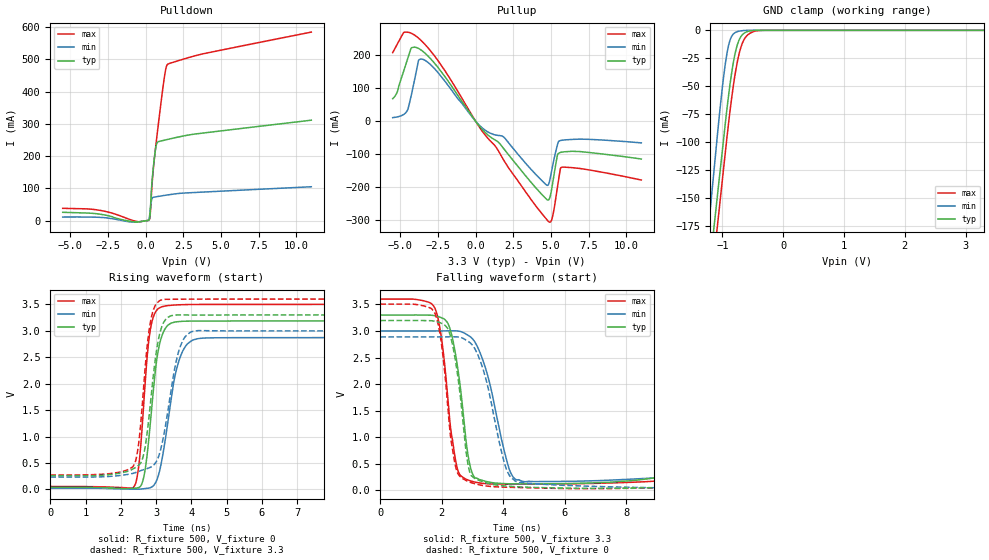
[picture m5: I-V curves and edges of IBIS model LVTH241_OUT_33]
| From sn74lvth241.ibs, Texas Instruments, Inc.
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[Model]   LVTH241_OUT_33
Model_type  3-state
Enable   Active-Low
Vref =   0
Rref =   500
Cref =   50p
Vmeas =   1.5
| variable   typ   min   max
C_comp   5.67pF   4.62pF   7.97pF
| C_pullup   4.93pF   0.26pF   7.08pF
| C_pulldown   9.55pF   2.16pF   32.43pF
| C_tri-state   5.67pF   4.62pF   7.97pF
[Temperature Range]   40   -40   100
| Ambient temperature   25   -40   85
[Voltage range]   3.3   3   3.6
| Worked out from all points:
|   slope of the pulldown table from 0 to 0.495 V, typ, clamps not added: 3.18 ohm
|   slope of the pullup table from 0 to 0.495 V, typ, clamps not added: 17.9 ohm
|   GND clamp passes 1 mA (typ) near -0.58 V on its own axis
|   rising waveform, R_fixture 500, V_fixture 0: 20-80 % time 295ps typ, 418ps min, 239ps max; typ from 0.041 V to 3.19 V
|   falling waveform, R_fixture 500, V_fixture 3.3: 20-80 % time 396ps typ, 676ps min, 378ps max; typ from 3.3 V to 0.26 V
|   rising waveform, R_fixture 500, V_fixture 3.3: 20-80 % time 323ps typ, 436ps min, 269ps max; typ from 0.261 V to 3.3 V
|   falling waveform, R_fixture 500, V_fixture 0: 20-80 % time 396ps typ, 675ps min, 384ps max; typ from 3.2 V to 0.041 V
[GND Clamp]
| LVTH241_OUT_33
|   Voltage   I(typ)   I(min)   I(max)
-5.5V     -2.862A    -3.036A    -2.907A
-1.245V   -228.9mA   -185.8mA   -258.5mA
-1.215V   -213.8mA   -168.6mA   -242.8mA
-1.175V   -193.8mA   -145.8mA   -222.1mA
-1.075V   -144mA     -89.2mA    -171mA
-925mV    -69.94mA   -20.46mA   -95.37mA
-875mV    -48.14mA   -8.719mA   -71.9mA
-800mV    -22.75mA   -2.299mA   -42.01mA
-725mV    -8.466mA   -746.4uA   -20.79mA
-650mV    -2.806mA   -185.7uA   -8.848mA
-310mV    -269.6nA   -70.47pA   -11.42uA
3.3V      32.83pA    25.31pA    1.688nA
[Pulldown]
| LVTH241_OUT_33
|   Voltage   I(typ)   I(min)   I(max)
-5.5V     25.99mA    11.41mA    38.31mA
-3.28V    21.76mA    10.81mA    33.9mA
-585mV    -3.904mA   -4.316mA   -2.507mA
215mV     1.677mA    2.589mA    1.896mA
305mV     26.06mA    31.6mA     17.21mA
425mV     118.9mA    68.07mA    110mA
580mV     192.7mA    73.06mA    190.3mA
710mV     233.6mA    74.11mA    244.7mA
1.225V    249.1mA    78.08mA    437.1mA
1.445V    251.5mA    79.68mA    483.5mA
3.79V     271.3mA    88.58mA    516.6mA
11V       311.3mA    105.1mA    584.1mA
[Pullup]
| LVTH241_OUT_33
|   Voltage   I(typ)   I(min)   I(max)
-5.5V     67.92mA    10.82mA    207.4mA
-4.615V   173.6mA    26.44mA    269.3mA
-4.28V    220.1mA    75.69mA    266.1mA
-3.79V    220mA      182.9mA    251.2mA
-3.465V   209.8mA    186.5mA    237.2mA
270mV     -15.96mA   -13.16mA   -19.22mA
1.855V    -82.19mA   -47.41mA   -116.7mA
4.89V     -235.3mA   -184.7mA   -304.8mA
5.11V     -188.9mA   -136.1mA   -288.5mA
5.435V    -102.2mA   -70.96mA   -199.1mA
5.69V     -93.81mA   -57.8mA    -139.6mA
11V       -114.3mA   -65.47mA   -177.8mA
[Ramp]
| LVTH241_OUT_33
| variable   typ   min   max
dV/dt_r   1.90/3.05E-10   1.72/4.25E-10   2.08/2.43E-10
dV/dt_f   1.91/4.19E-10   1.70/6.99E-10   2.09/4.01E-10
R_load = 500
[Rising Waveform]
| LVTH241_OUT_33
R_fixture =   500
C_fixture =   0
L_fixture =   0
V_fixture =   0
V_fixture_min = 0
V_fixture_max = 0
|   Time   V(typ)   V(min)   V(max)
0s        41.42mV    24.68mV    57.22mV
2.37ns    22.92mV    5.962mV    52.35mV
2.5ns     34.94mV    6.563mV    403.8mV
2.635ns   192.6mV    13.04mV    1.48V
2.845ns   1.324V     36.48mV    3.056V
3.055ns   2.609V     247.2mV    3.417V
3.33ns    3.103V     1.262V     3.476V
3.73ns    3.179V     2.583V     3.494V
4.365ns   3.184V     2.864V     3.498V
50ns      3.188V     2.873V     3.5V
[Falling Waveform]
| LVTH241_OUT_33
R_fixture =   500
C_fixture =   0
L_fixture =   0
V_fixture =   3.3
V_fixture_min = 3
V_fixture_max = 3.6
|   Time   V(typ)   V(min)   V(max)
0s        3.3V       3V         3.6V
1.74ns    3.29V      3.001V     3.463V
1.965ns   3.255V     3.001V     2.962V
2.19ns    3.152V     3.002V     1.773V
2.535ns   2.233V     2.998V     357.2mV
2.91ns    486mV      2.898V     185.2mV
3.295ns   194.3mV    2.514V     136.4mV
4.19ns    126mV      402.3mV    119.3mV
4.68ns    122.7mV    165.1mV    119.8mV
50ns      260.2mV    234.4mV    273mV
[Rising Waveform]
| LVTH241_OUT_33
R_fixture =   500
C_fixture =   0
L_fixture =   0
V_fixture =   3.3
V_fixture_min = 3
V_fixture_max = 3.6
|   Time   V(typ)   V(min)   V(max)
0s        260.8mV    234.8mV    273.4mV
2.34ns    386.3mV    303.9mV    428.1mV
2.495ns   454.3mV    339.1mV    820.4mV
2.63ns    618.6mV    370.9mV    1.794V
2.845ns   1.671V     421.7mV    3.189V
3.05ns    2.782V     587.6mV    3.541V
3.265ns   3.211V     1.211V     3.595V
3.67ns    3.301V     2.677V     3.597V
4.195ns   3.298V     3.004V     3.599V
50ns      3.3V       3V         3.6V
[Falling Waveform]
| LVTH241_OUT_33
R_fixture =   500
C_fixture =   0
L_fixture =   0
V_fixture =   0
V_fixture_min = 0
V_fixture_max = 0
|   Time   V(typ)   V(min)   V(max)
0s        3.196V     2.888V     3.505V
1.74ns    3.186V     2.888V     3.366V
1.965ns   3.151V     2.889V     2.852V
2.185ns   3.05V      2.89V      1.639V
2.47ns    2.343V     2.889V     402mV
2.895ns   371.6mV    2.788V     161.5mV
3.515ns   132.1mV    1.904V     80mV
4.15ns    80.49mV    333.4mV    60.1mV
5.015ns   57.2mV     125mV      48.23mV
50ns      41.43mV    24.68mV    57.29mV
